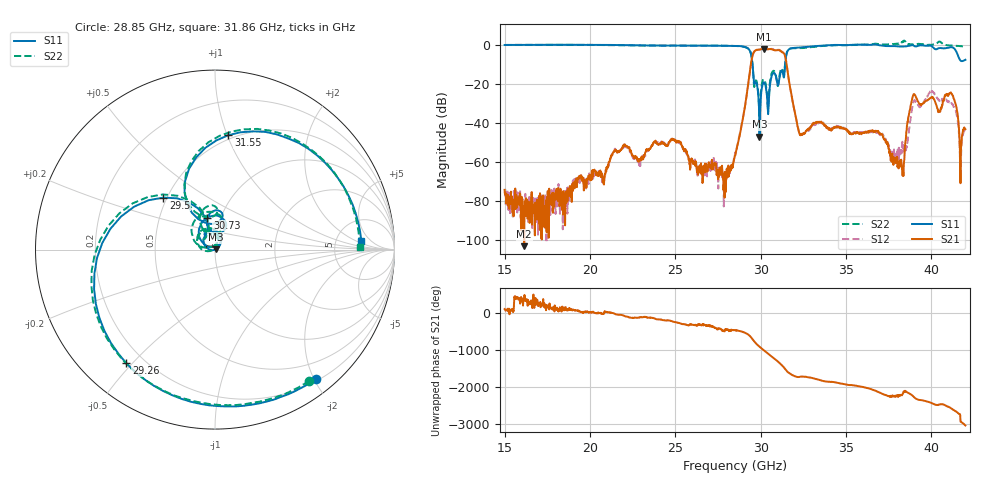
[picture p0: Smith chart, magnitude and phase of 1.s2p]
!The following data was pulled from an Agilent PNA
!This sNp file was generated from the data in the RF Test software
!NOTE:  Smoothing/Math/Corrections applied on any given trace ARE included in the data saved here
# MHz S dB R 50
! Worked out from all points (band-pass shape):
!   1601 points, 15 GHz to 42 GHz, reference 50 ohm
!   highest |S21| = -2.15 dB at 30.17 GHz (marker M1); lowest = -103.0 dB at 16.15 GHz (marker M2)
!   |S21| within 3 dB of the highest: 29.54 GHz to 31.41 GHz (1.866 GHz wide, 6.12 % of centre)
!   lowest |S11| = -47.0 dB at 29.93 GHz (marker M3), VSWR 1.01, Z = 50.4 + j0.269 ohm
!   |S11| at or under -10 dB: 29.52 GHz to 31.44 GHz (1.917 GHz wide, 6.29 % of centre)
!   |S22| runs from -42.9 to 2.1 dB; largest |S21 - S12| = 0.038
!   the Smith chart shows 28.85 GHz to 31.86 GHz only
!   S11 on the Smith chart (normalised r, x): 28.85 GHz: 0.24, -2.03; 29.26 GHz: 0.13, -0.48; 29.5 GHz: 0.48, +0.33; 30.73 GHz: 0.86, +0.32; 31.55 GHz: 0.47, +1.01; 31.86 GHz: 9.18, +2.65
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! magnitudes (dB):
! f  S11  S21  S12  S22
! 15 GHz  -0.2  -74.2  -75.6  -0.1
! 16.15 GHz  -0.1  -103.0  -83.6  -0.1
! 19.51 GHz  -0.1  -67.6  -68.8  -0.1
! 24.01 GHz  -0.5  -51.3  -50.6  -0.5
! 27.88 GHz  -0.6  -71.4  -75.1  -0.5
! 28.5 GHz  -0.6  -56.7  -55.7  -0.7
! 28.85 GHz  -0.8  -42.7  -42.1  -0.9
! 29.26 GHz  -1.9  -20.7  -21.6  -1.9
! 29.5 GHz  -7.8  -6.5  -7.0  -7.5
! 29.93 GHz  -47.0  -2.5  -2.6  -42.9
! 30.17 GHz  -19.2  -2.2  -2.1  -17.7
! 30.73 GHz  -14.7  -2.6  -2.5  -13.5
! 31.55 GHz  -3.9  -11.8  -12.0  -3.5
! 31.86 GHz  -1.8  -28.2  -28.4  -1.8
! 32.33 GHz  -1.4  -46.3  -46.0  -1.8
! 33.01 GHz  -0.9  -41.2  -41.8  -1.2
! 37.51 GHz  -0.8  -53.2  -52.3  0.1
! 38.3 GHz  -1.0  -62.8  -49.6  1.3
! 39 GHz  -0.6  -25.3  -28.5  0.1
! 41.14 GHz  -1.3  -24.4  -29.4  -0.5
! 41.71 GHz  -8.2  -70.8  -69.0  -0.8
! 42 GHz  -7.7  -43.2  -44.0  -1.1
